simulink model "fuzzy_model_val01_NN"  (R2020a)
settings: Solver=VariableStepAuto  StartTime=0.0  StopTime=tfin  RelTol=1e-3
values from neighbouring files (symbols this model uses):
  Ts = 5    [sisopres.m]
undefined symbols (not defined in the file or in its folder): magnitude
libraries: neural x10

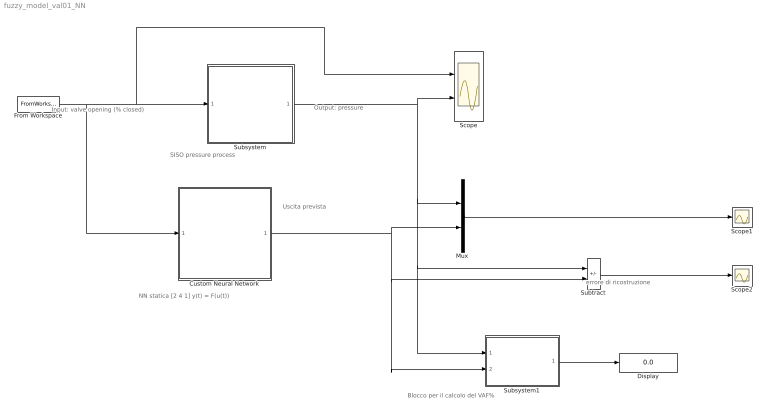
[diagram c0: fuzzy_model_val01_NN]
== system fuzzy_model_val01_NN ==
  note: Blocco per il calcolo del VAF%
  note: errore di ricostruzione
  note: Uscita prevista
  note: NN statica [2 4 1] y(t) = F(u(t))
  note: Output: pressure
  note: Input: valve opening (% closed)
  note: SISO pressure process
  Custom Neural Network : Subsystem
      mask help: Custom Neural Network
  Display : Display
  From Workspace : FromWorkspace  VariableName=[tsim U]  SampleTime=Ts
  Mux : Mux  Inputs=2
  Scope : Scope  NumInputPorts=2
  Scope1 : Scope
  Scope2 : Scope
  Subsystem : Subsystem
  Subsystem1 : Subsystem
  Subtract : Sum  Inputs=+-
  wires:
  From Workspace/1 -> Custom Neural Network/1(Input), Scope/1, Subsystem/1(u)
  Mux/1 -> Scope1/1
  Subtract/1 -> Scope2/1
  Custom Neural Network/1(Output) -> Subsystem1/2(y_prev), Subtract/2, Mux/2
  Subsystem/1(y) -> Subsystem1/1(y_mis), Subtract/1, Mux/1, Scope/2
  Subsystem1/1(VAF%) -> Display/1

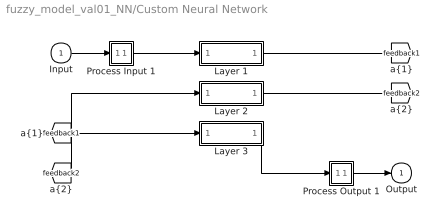
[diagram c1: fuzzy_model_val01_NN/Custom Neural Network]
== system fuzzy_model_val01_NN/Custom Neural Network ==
  Input : Inport  PortDimensions=1  SampleTime=5
  Layer 1 : Subsystem
  Layer 2 : Subsystem
  Layer 3 : Subsystem
  Process Input 1 : Subsystem
  Process Output 1 : Subsystem
  Output : Outport  InitialOutput=0
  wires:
  Input/1 -> Process Input 1/1(x)
  Process Output 1/1(y) -> Output/1
  Process Input 1/1(p) -> Layer 1/1("p{1}")
  Layer 1/1("a{1}") -> [feedback1]
  [feedback1] -> Layer 2/1("a{1} ")
  Layer 2/1("a{2}") -> [feedback2]
  [feedback2] -> Layer 3/1("a{2} ")
  Layer 3/1("a{3}") -> Process Output 1/1(a)

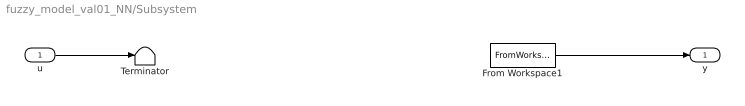
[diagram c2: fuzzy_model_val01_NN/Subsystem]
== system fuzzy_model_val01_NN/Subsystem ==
  u : Inport
  From Workspace1 : FromWorkspace  VariableName=[tsim Y]  SampleTime=Ts
  Terminator : Terminator
  y : Outport
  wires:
  From Workspace1/1 -> y/1
  u/1 -> Terminator/1

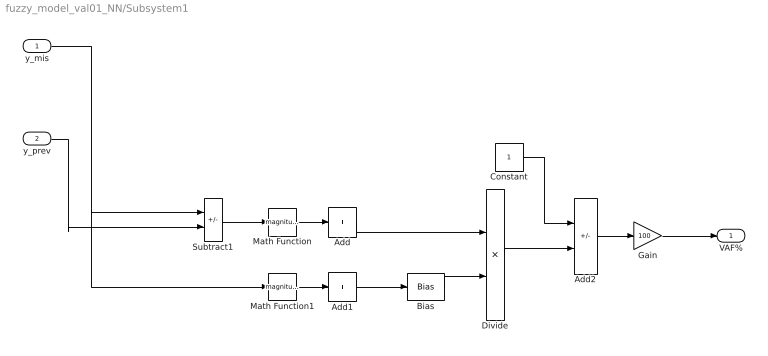
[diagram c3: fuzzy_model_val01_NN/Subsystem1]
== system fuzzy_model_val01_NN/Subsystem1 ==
  y_mis : Inport
  y_prev : Inport  Port=2
  Add : Sum  Inputs=+
  Add1 : Sum  Inputs=+
  Add2 : Sum  Inputs=+-
  Bias : Bias  Bias=1e-7
  Constant : Constant
  Divide : Product  Inputs=*/
  Gain : Gain  Gain=100
  Math Function : Math  Operator=magnitude^2
  Math Function1 : Math  Operator=magnitude^2
  Subtract1 : Sum  Inputs=+-
  VAF% : Outport
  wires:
  Add2/1 -> Gain/1
  Math Function/1 -> Add/1
  Bias/1 -> Divide/2
  y_mis/1 -> Math Function1/1, Subtract1/1
  Add1/1 -> Bias/1
  Math Function1/1 -> Add1/1
  Subtract1/1 -> Math Function/1
  Constant/1 -> Add2/1
  Divide/1 -> Add2/2
  Add/1 -> Divide/1
  y_prev/1 -> Subtract1/2
  Gain/1 -> VAF%/1

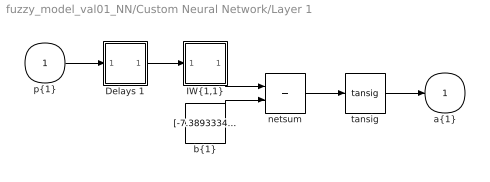
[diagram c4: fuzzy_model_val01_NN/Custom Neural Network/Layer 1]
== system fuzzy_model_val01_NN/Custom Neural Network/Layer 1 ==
  "p{1}" : Inport  PortDimensions=1  SampleTime=5
  Delays 1 : Subsystem
  "IW{1,1}" : Subsystem
  "b{1}" : Constant  Value=[-7.38933347823103048312987084500491619110107421875;-3.186102848194679371118809285690076649188995361328125]
  netsum : Sum  Inputs=2  InputSameDT=on  SaturateOnIntegerOverflow=on
  tansig : neural/Transfer Functions/tansig
  "a{1}" : Outport  InitialOutput=[0;0]
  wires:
  "p{1}"/1 -> Delays 1/1("p{1}")
  Delays 1/1("pd{1,1}") -> "IW{1,1}"/1("pd{1,1}")
  "IW{1,1}"/1("iz{1,1}") -> netsum/1
  "b{1}"/1 -> netsum/2
  netsum/1 -> tansig/1
  tansig/1 -> "a{1}"/1

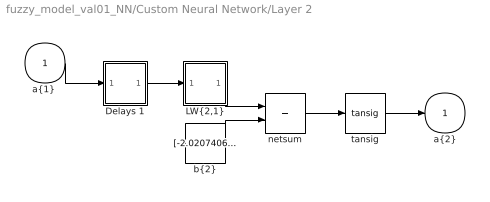
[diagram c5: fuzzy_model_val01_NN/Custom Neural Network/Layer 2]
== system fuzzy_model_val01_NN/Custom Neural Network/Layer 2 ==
  "a{1} " : Inport  PortDimensions=2  SampleTime=5
  Delays 1 : Subsystem
  "LW{2,1}" : Subsystem
  "b{2}" : Constant  Value=[-2.0207406085147141538982396014034748077392578125;-0.84306008052592995571927758646779693663120269775390625;1.3883331548319810533342888447805307805538177490234375;-2.84540676308034345964870226453058421611785888671875]
  netsum : Sum  Inputs=2  InputSameDT=on  SaturateOnIntegerOverflow=on
  tansig : neural/Transfer Functions/tansig
  "a{2}" : Outport  InitialOutput=[0;0;0;0]
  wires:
  "a{1} "/1 -> Delays 1/1("p{2}")
  Delays 1/1("pd{2,1}") -> "LW{2,1}"/1("ad{2,1}")
  "LW{2,1}"/1("lz{2,1}") -> netsum/1
  "b{2}"/1 -> netsum/2
  netsum/1 -> tansig/1
  tansig/1 -> "a{2}"/1

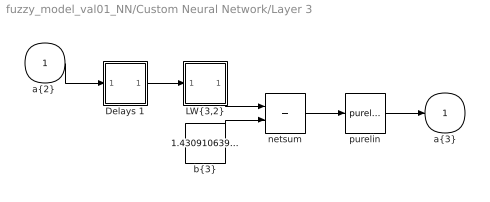
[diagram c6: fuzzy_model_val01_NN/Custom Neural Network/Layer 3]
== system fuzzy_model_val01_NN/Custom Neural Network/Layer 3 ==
  "a{2} " : Inport  PortDimensions=4  SampleTime=5
  Delays 1 : Subsystem
  "LW{3,2}" : Subsystem
  "b{3}" : Constant  Value=1.4309106391766761579020794670213945209980010986328125
  netsum : Sum  Inputs=2  InputSameDT=on  SaturateOnIntegerOverflow=on
  purelin : neural/Transfer Functions/purelin
  "a{3}" : Outport  InitialOutput=0
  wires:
  "a{2} "/1 -> Delays 1/1("p{3}")
  Delays 1/1("pd{3,2}") -> "LW{3,2}"/1("ad{3,2}")
  "LW{3,2}"/1("lz{3,2}") -> netsum/1
  "b{3}"/1 -> netsum/2
  netsum/1 -> purelin/1
  purelin/1 -> "a{3}"/1

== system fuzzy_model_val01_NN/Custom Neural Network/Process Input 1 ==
  x : Inport  PortDimensions=1  SampleTime=5
  p : Outport  PortDimensions=1  SampleTime=5
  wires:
  x/1 -> p/1

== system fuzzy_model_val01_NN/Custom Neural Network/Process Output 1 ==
  a : Inport  PortDimensions=1  SampleTime=5
  y : Outport  PortDimensions=1  SampleTime=5
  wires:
  a/1 -> y/1

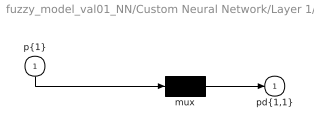
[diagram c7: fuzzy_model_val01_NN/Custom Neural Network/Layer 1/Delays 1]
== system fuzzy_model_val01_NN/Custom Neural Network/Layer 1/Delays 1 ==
  "p{1}" : Inport  PortDimensions=1  SampleTime=5
  mux : Mux  Inputs=1
  "pd{1,1}" : Outport
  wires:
  "p{1}"/1 -> mux/1
  mux/1 -> "pd{1,1}"/1

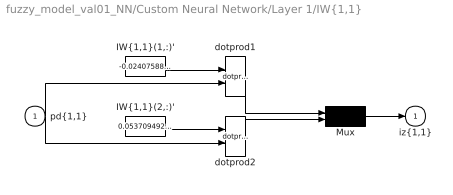
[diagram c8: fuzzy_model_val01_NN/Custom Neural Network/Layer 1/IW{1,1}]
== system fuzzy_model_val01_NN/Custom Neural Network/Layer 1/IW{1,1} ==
  "pd{1,1}" : Inport  PortDimensions=1  SampleTime=5
  "IW{1,1}(1,:)'" : Constant  Value=-0.0240758877335825079157860528766832430846989154815673828125
  "IW{1,1}(2,:)'" : Constant  Value=0.05370949299328446613355225736086140386760234832763671875
  Mux : Mux  Inputs=2
  dotprod1 : neural/Weight Functions/dotprod
  dotprod2 : neural/Weight Functions/dotprod
  "iz{1,1}" : Outport
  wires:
  "IW{1,1}(1,:)'"/1 -> dotprod1/1
  "pd{1,1}"/1 -> dotprod1/2, dotprod2/2
  dotprod1/1 -> Mux/1
  "IW{1,1}(2,:)'"/1 -> dotprod2/1
  dotprod2/1 -> Mux/2
  Mux/1 -> "iz{1,1}"/1

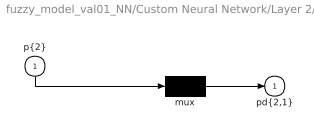
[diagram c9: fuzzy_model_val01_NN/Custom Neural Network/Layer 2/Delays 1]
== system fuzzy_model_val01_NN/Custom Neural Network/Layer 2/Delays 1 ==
  "p{2}" : Inport  PortDimensions=2  SampleTime=5
  mux : Mux  Inputs=1
  "pd{2,1}" : Outport
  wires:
  "p{2}"/1 -> mux/1
  mux/1 -> "pd{2,1}"/1

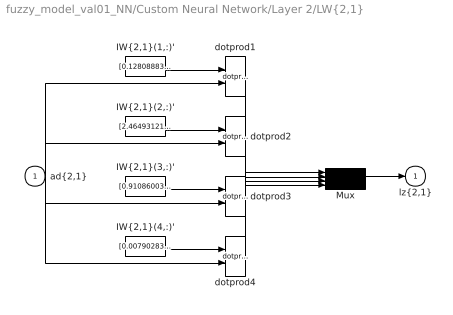
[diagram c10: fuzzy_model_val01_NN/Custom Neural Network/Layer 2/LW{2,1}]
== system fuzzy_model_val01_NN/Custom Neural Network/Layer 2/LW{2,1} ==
  "ad{2,1}" : Inport  PortDimensions=2  SampleTime=5
  "IW{2,1}(1,:)'" : Constant  Value=[0.128088837215155848525682813487946987152099609375;4.4068035339317219722943264059722423553466796875]
  "IW{2,1}(2,:)'" : Constant  Value=[2.464931216039210948309801096911542117595672607421875;1.208959818472298053393387817777693271636962890625]
  "IW{2,1}(3,:)'" : Constant  Value=[0.91086003469910503671513879453414119780063629150390625;2.75364517606309533448438742198050022125244140625]
  "IW{2,1}(4,:)'" : Constant  Value=[0.00790283586035346423404046589666904765181243419647216796875;-2.790030115785254505311741013429127633571624755859375]
  Mux : Mux
  dotprod{1..4} (4 alike) : neural/Weight Functions/dotprod
  "lz{2,1}" : Outport
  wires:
  "IW{2,1}(1,:)'"/1 -> dotprod1/1
  "ad{2,1}"/1 -> dotprod1/2, dotprod2/2, dotprod3/2, dotprod4/2
  dotprod1/1 -> Mux/1
  "IW{2,1}(2,:)'"/1 -> dotprod2/1
  dotprod2/1 -> Mux/2
  "IW{2,1}(3,:)'"/1 -> dotprod3/1
  dotprod3/1 -> Mux/3
  "IW{2,1}(4,:)'"/1 -> dotprod4/1
  dotprod4/1 -> Mux/4
  Mux/1 -> "lz{2,1}"/1

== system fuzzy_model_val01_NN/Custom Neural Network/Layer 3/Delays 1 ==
  "p{3}" : Inport  PortDimensions=4  SampleTime=5
  mux : Mux  Inputs=1
  "pd{3,2}" : Outport
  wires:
  "p{3}"/1 -> mux/1
  mux/1 -> "pd{3,2}"/1

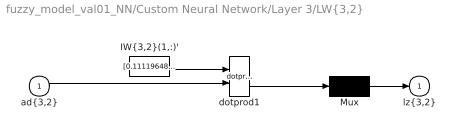
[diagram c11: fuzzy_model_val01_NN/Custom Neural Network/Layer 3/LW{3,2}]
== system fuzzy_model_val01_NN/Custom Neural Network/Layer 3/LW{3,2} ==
  "ad{3,2}" : Inport  PortDimensions=4  SampleTime=5
  "IW{3,2}(1,:)'" : Constant  Value=[0.1111964810748821974595301753652165643870830535888671875;0.153274542893776233309921508407569490373134613037109375;0.044172991137541479933492638565439847297966480255126953125;-0.07327769964756190856913775633074692450463771820068359375]
  Mux : Mux  Inputs=1
  dotprod1 : neural/Weight Functions/dotprod
  "lz{3,2}" : Outport
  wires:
  "IW{3,2}(1,:)'"/1 -> dotprod1/1
  "ad{3,2}"/1 -> dotprod1/2
  dotprod1/1 -> Mux/1
  Mux/1 -> "lz{3,2}"/1
